(* Logix 5000 Rung export; software revision 16.03 *)

MODULES
   MCMR : vendor None type None code None
   Remote_ENBT : vendor None type None code None
END_MODULES

TYPE MCMRInitOutputData :   // Used to bring the Module into a known state after a restart operation.
STRUCT
   InitOutBlkIDLim : INT;   // Block Index Limit for ReadData size of the array
END_STRUCT
END_TYPE

TYPE MCMRCmdControl :   // Tags for command control
STRUCT
   CmdTrigger : BOOL;   // Command Trigger
   CmdControlData : INT[21];   // Command Control Data
   CmdControlResp : INT[5];   // Command Control Response
   CmdErrTrigger : BOOL;   // Command Error Trigger
   CmdErrData : INT[102];   // Command Error Data
END_STRUCT
END_TYPE

TYPE MCMRDATA :   // This object contains the Read & Write Data Arrays.
STRUCT
   ReadData : INT[600];   // Data read from module
   WriteData : INT[600];   // Data to write to module
END_STRUCT
END_TYPE

TYPE MCMRUTIL :   // This object stores all the variables required for data transfer operation between the module and the controller.
STRUCT
   LastRead : INT;   // Index of last read block
   LastWrite : INT;   // Index of last write block
   BlockIndex : INT;   // Computed block offset for data table
   ReadDataSize : DINT;   // Size of Read Data Array
   WriteDataSize : DINT;   // Size of Write Data Array
   RBTSremainder : INT;   // Computed remainder from Read Data Array size
   WBTSremainder : INT;   // Computed remainder from Write Data Array size
   MaxReadBlock : DINT;   // Maximum read block
   MaxWriteBlock : DINT;   // Maximum write block
   InitOutputData : MCMRInitOutputData;   // This is to initialize output data module reads data from PLC
END_STRUCT
END_TYPE

TYPE MCMRModuleDef :   // This object contains variables to be used with the module and status data related to the module.
STRUCT
   DATA : MCMRDATA;   // Read Data and Write Data
   STATUS : MCMRSTATUS;   // Status information in each read block
   CONTROL : MCMRCONTROL;   // Command Control Object
   UTIL : MCMRUTIL;   // Backplane Object
END_STRUCT
END_TYPE

TYPE MCMRSTATUS :   // This status data is returned on each read block and can be used to detect proper module operation.
STRUCT
   PassCnt : INT;   // Program cycle counter
   Product : INT[2];   // Product Name
   Rev : INT[2];   // Revision Level Number
   OP : INT[2];   // Operating Level Number
   Run : INT[2];   // Run Number
   Port1Stats : MCMRPortStats;   // Port error statistics for Port 1
   Port2Stats : MCMRPortStats;   // Port error statistics for Port 2
   Block : MCMRBlockStats;   // Block transfer statistics
   Port1CurrentErr : INT;   // Current error/index for Port 1
   Port1LastErr : INT;   // Last error/index for Port 1
   Port2CurrentErr : INT;   // Current error/index for Port 2
   Port2LastErr : INT;   // Last error/index for Port 2
   StatusMsgData : INT[46];   // Triggers status message data
   StatusTrigger : BOOL;   // Triggers Status reading.
END_STRUCT
END_TYPE

TYPE MCMRCONTROL :   // Tags used for special blocks
STRUCT
   ColdBoot : BOOL;   // Cold Boot
   WarmBoot : BOOL;   // Warm Boot
   CmdControlP1 : MCMRCmdControl;   // Command Control for Port 1
   CmdControlP2 : MCMRCmdControl;   // Command Control for Port 2
   EventTriggerP1 : BOOL;   // Triggers the Event Command.
   EventTriggerP2 : BOOL;   // Triggers the Event Command.
   EventCmdP1 : MCMREventCmd[100];   // Event Command for Port 1
   EventCmdP2 : MCMREventCmd[100];   // Event Command for Port 2
   EventCmdRespP1 : INT[5];   // Event Command Response for Port 1
   EventCmdRespP2 : INT[5];   // Event Command Response for Port 2
END_STRUCT
END_TYPE

TYPE MCMREventCmd :   // This object is used to contain the attributes to define a master command. An array of these objects is used for each port.
STRUCT
   Enable : INT;   // 0=Disable,1=Continuous,2=Event Command
   IntAddress : INT;   // Module's internal address associated with the command
   PollInt : INT;   // Minimum number of seconds between issuance of command (0-65535 Sec)
   Count : INT;   // Number of registers associated with the command
   Swap : INT;   // Swap code used with command
   Device : INT;   // Device index in Device Table to associate with the command
   Func : INT;   // Function code for the command
   DevAddress : INT;   // Address in device associated with the command
END_STRUCT
END_TYPE

TYPE MCMRPortStats :   // This object is used to store the port statistics
STRUCT
   PortTrigger : BOOL;   // Triggers port status reading
   CmdReq : INT;   // Total number of command list requests sent
   CmdResp : INT;   // Total number of command list responses received
   CmdErr : INT;   // Total number of command list errors
   Requests : INT;   // Total number of requests for port
   Responses : INT;   // Total number of responses for port
   ErrSent : INT;   // Total number of errors sent
   ErrRec : INT;   // Total number of errors received
   SlaveStats : SINT[250];   // Port Slave status values
END_STRUCT
END_TYPE

TYPE MCMRBlockStats :   // This object is used to store the block transfer statistics for the module.
STRUCT
   Read : INT;   // Total number of read block transfers
   Write : INT;   // Total number of write block transfers
   Parse : INT;   // Total number of blocks parsed
   Event : INT;   // Total number of event blocks received
   Cmd : INT;   // Total number of command blocks received
   Err : INT;   // Total number of block transfer errors
END_STRUCT
END_TYPE

ADD_ON_INSTRUCTION AOI56MCMR   (* revision 1.5, vendor ProSoft Technology Inc., ExecutePrescan *)
// Add-On - MVI56-MCMR & MVI56E-MCMR modules.
// Revision note:
// v1.5 - Initialize output data block now flexible to accommodate for flexible read and write data arrays.
VAR_IN_OUT
   Connection_Input : INT[42]; {required}   // Input parameters.
   Connection_Output : INT[42]; {required}   // Output parameters.
   MCMR : MCMRModuleDef; {required}
   CmdControlP1_MSG : MESSAGE; {required}
   CmdControlP2_MSG : MESSAGE; {required}
   CmdControlRespP1_MSG : MESSAGE; {required}
   CmdControlRespP2_MSG : MESSAGE; {required}
   CmdErrorP1_MSG : MESSAGE; {required}
   CmdErrorP2_MSG : MESSAGE; {required}
   EventCmdP1_MSG : MESSAGE; {required}
   EventCmdP2_MSG : MESSAGE; {required}
   EventCmdRespP1_MSG : MESSAGE; {required}
   EventCmdRespP2_MSG : MESSAGE; {required}
   SlaveStatusP1_MSG : MESSAGE; {required}
   SlaveStatusP2_MSG : MESSAGE; {required}
   ModuleStatus_MSG : MESSAGE; {required}
END_VAR
VAR
   MJFAULTS : DINT[12];
END_VAR

ROUTINE Logic   (* ladder *)
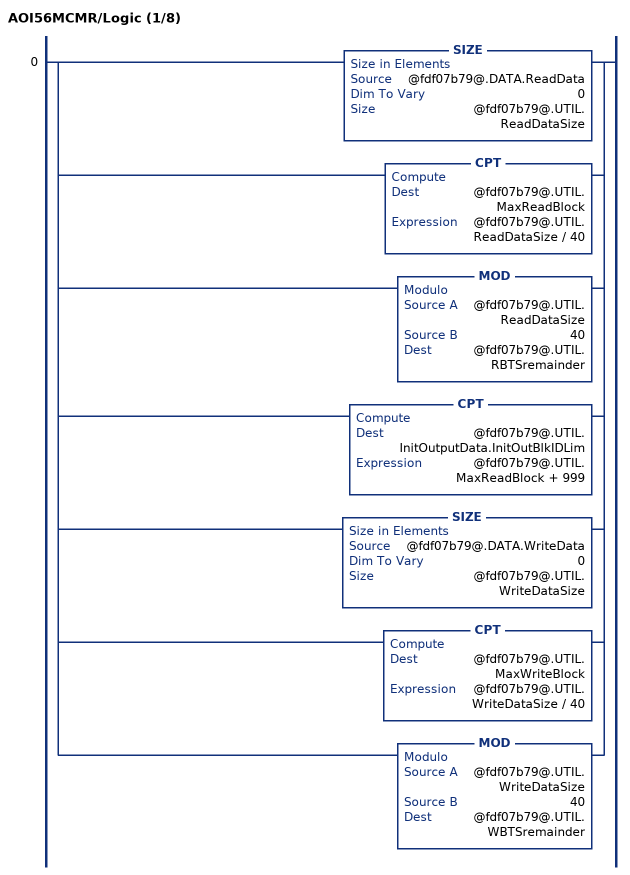
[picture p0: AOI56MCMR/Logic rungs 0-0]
   0: [SIZE(@fdf07b79@.DATA.ReadData,0,@fdf07b79@.UTIL.ReadDataSize) ,CPT(@fdf07b79@.UTIL.MaxReadBlock,@fdf07b79@.UTIL.ReadDataSize / 40) ,MOD(@fdf07b79@.UTIL.ReadDataSize,40,@fdf07b79@.UTIL.RBTSremainder) ,CPT(@fdf07b79@.UTIL.InitOutputData.InitOutBlkIDLim,@fdf07b79@.UTIL.MaxReadBlock + 999) ,SIZE(@fdf07b79@.DATA.WriteData,0,@fdf07b79@.UTIL.WriteDataSize) ,CPT(@fdf07b79@.UTIL.MaxWriteBlock,@fdf07b79@.UTIL.WriteDataSize / 40) ,MOD(@fdf07b79@.UTIL.WriteDataSize,40,@fdf07b79@.UTIL.WBTSremainder) ];
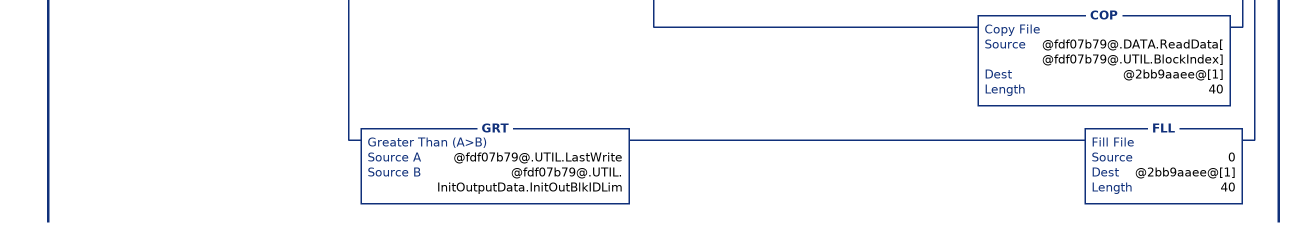
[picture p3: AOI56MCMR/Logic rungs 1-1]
   // This rung is used to check for a new read block from the MVI56-MBP module in slot 1.  If new data is available, the LastRead and word[0] will not be equal.  This will force the program to call the ReadData subroutine to process the new data received.  After the new data is placed in the Modbus Data Table, the program will send new data to the module using the WriteData subroutine.
   1: NEQ(@de25fda7@[41],@fdf07b79@.UTIL.LastRead)[MOV(@de25fda7@[41],@fdf07b79@.UTIL.LastRead) ,GEQ(@fdf07b79@.UTIL.LastRead,1) [LEQ(@fdf07b79@.UTIL.LastRead,@fdf07b79@.UTIL.MaxReadBlock) [CPT(@fdf07b79@.UTIL.BlockIndex,(@fdf07b79@.UTIL.LastRead - 1) * 40) ,COP(@de25fda7@[1],@fdf07b79@.DATA.ReadData[@fdf07b79@.UTIL.BlockIndex],40) ] ,CMP(@fdf07b79@.UTIL.LastRead - @fdf07b79@.UTIL.MaxReadBlock = 1) GRT(@fdf07b79@.UTIL.RBTSremainder,0) [CPT(@fdf07b79@.UTIL.BlockIndex,(@fdf07b79@.UTIL.LastRead - 1) * 40) ,COP(@de25fda7@[1],@fdf07b79@.DATA.ReadData[@fdf07b79@.UTIL.BlockIndex],@fdf07b79@.UTIL.RBTSremainder) ] ] ,MOV(@de25fda7@[0],@fdf07b79@.UTIL.LastWrite) ,XIC(@fdf07b79@.CONTROL.WarmBoot) [MOV(9998,@fdf07b79@.UTIL.LastWrite) ,MOV(9998,@2bb9aaee@[0]) ,OTU(@fdf07b79@.CONTROL.WarmBoot) ] ,XIC(@fdf07b79@.CONTROL.ColdBoot) [MOV(9999,@fdf07b79@.UTIL.LastWrite) ,MOV(9999,@2bb9aaee@[0]) ,OTU(@fdf07b79@.CONTROL.ColdBoot) ] ,[EQU(-1,@fdf07b79@.UTIL.LastWrite) ,EQU(0,@fdf07b79@.UTIL.LastWrite) ] MOV(@fdf07b79@.UTIL.LastWrite,@2bb9aaee@[0]) ,GEQ(@fdf07b79@.UTIL.LastWrite,1) [LEQ(@fdf07b79@.UTIL.LastWrite,@fdf07b79@.UTIL.MaxWriteBlock) [CPT(@fdf07b79@.UTIL.BlockIndex,(@fdf07b79@.UTIL.LastWrite - 1) * 40) ,COP(@fdf07b79@.DATA.WriteData[@fdf07b79@.UTIL.BlockIndex],@2bb9aaee@[1],40) ] ,CMP(@fdf07b79@.UTIL.LastWrite - @fdf07b79@.UTIL.MaxWriteBlock = 1) GRT(@fdf07b79@.UTIL.WBTSremainder,0) [CPT(@fdf07b79@.UTIL.BlockIndex,(@fdf07b79@.UTIL.LastWrite - 1) * 40) ,COP(@fdf07b79@.DATA.WriteData[@fdf07b79@.UTIL.BlockIndex],@2bb9aaee@[1],@fdf07b79@.UTIL.WBTSremainder) ] ,MOV(@fdf07b79@.UTIL.LastWrite,@2bb9aaee@[0]) ] ,LIM(1000,@fdf07b79@.UTIL.LastWrite,1124) [LEQ(@fdf07b79@.UTIL.LastWrite,@fdf07b79@.UTIL.InitOutputData.InitOutBlkIDLim) [CPT(@fdf07b79@.UTIL.BlockIndex,(@fdf07b79@.UTIL.LastWrite - 1000) * 40) ,COP(@fdf07b79@.DATA.ReadData[@fdf07b79@.UTIL.BlockIndex],@2bb9aaee@[1],40) ] ,GRT(@fdf07b79@.UTIL.LastWrite,@fdf07b79@.UTIL.InitOutputData.InitOutBlkIDLim) FLL(0,@2bb9aaee@[1],40) ] ];
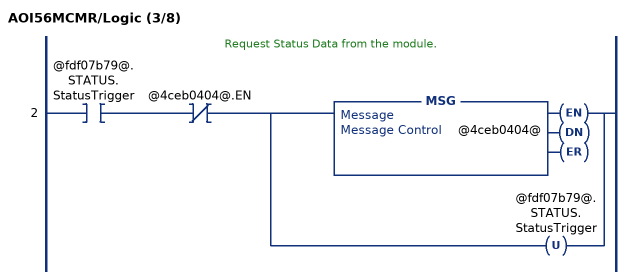
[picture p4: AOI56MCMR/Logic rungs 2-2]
   // Request Status Data from the module.
   2: XIC(@fdf07b79@.STATUS.StatusTrigger)XIO(@4ceb0404@.EN)[MSG(@4ceb0404@) ,OTU(@fdf07b79@.STATUS.StatusTrigger) ];
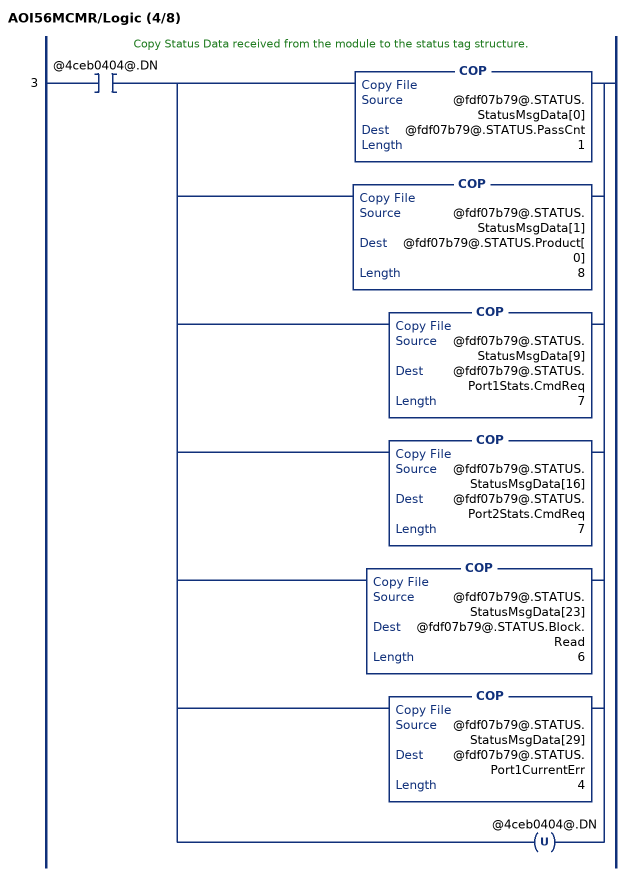
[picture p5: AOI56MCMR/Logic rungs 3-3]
   // Copy Status Data received from the module to the status tag structure.
   3: XIC(@4ceb0404@.DN)[COP(@fdf07b79@.STATUS.StatusMsgData[0],@fdf07b79@.STATUS.PassCnt,1) ,COP(@fdf07b79@.STATUS.StatusMsgData[1],@fdf07b79@.STATUS.Product[0],8) ,COP(@fdf07b79@.STATUS.StatusMsgData[9],@fdf07b79@.STATUS.Port1Stats.CmdReq,7) ,COP(@fdf07b79@.STATUS.StatusMsgData[16],@fdf07b79@.STATUS.Port2Stats.CmdReq,7) ,COP(@fdf07b79@.STATUS.StatusMsgData[23],@fdf07b79@.STATUS.Block.Read,6) ,COP(@fdf07b79@.STATUS.StatusMsgData[29],@fdf07b79@.STATUS.Port1CurrentErr,4) ,OTU(@4ceb0404@.DN) ];
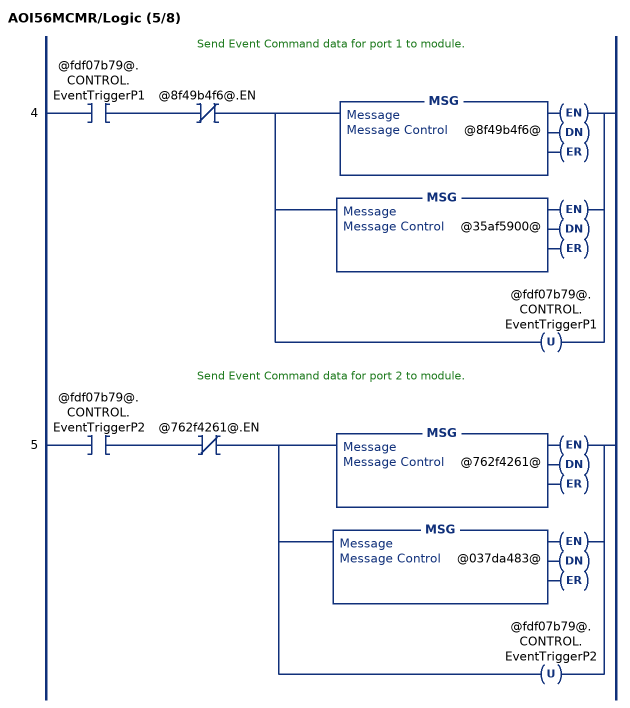
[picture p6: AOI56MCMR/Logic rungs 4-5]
   // Send Event Command data for port 1 to module.
   4: XIC(@fdf07b79@.CONTROL.EventTriggerP1)XIO(@8f49b4f6@.EN)[[MSG(@8f49b4f6@) ,MSG(@35af5900@) ] ,OTU(@fdf07b79@.CONTROL.EventTriggerP1) ];
   // Send Event Command data for port 2 to module.
   5: XIC(@fdf07b79@.CONTROL.EventTriggerP2)XIO(@762f4261@.EN)[[MSG(@762f4261@) ,MSG(@037da483@) ] ,OTU(@fdf07b79@.CONTROL.EventTriggerP2) ];
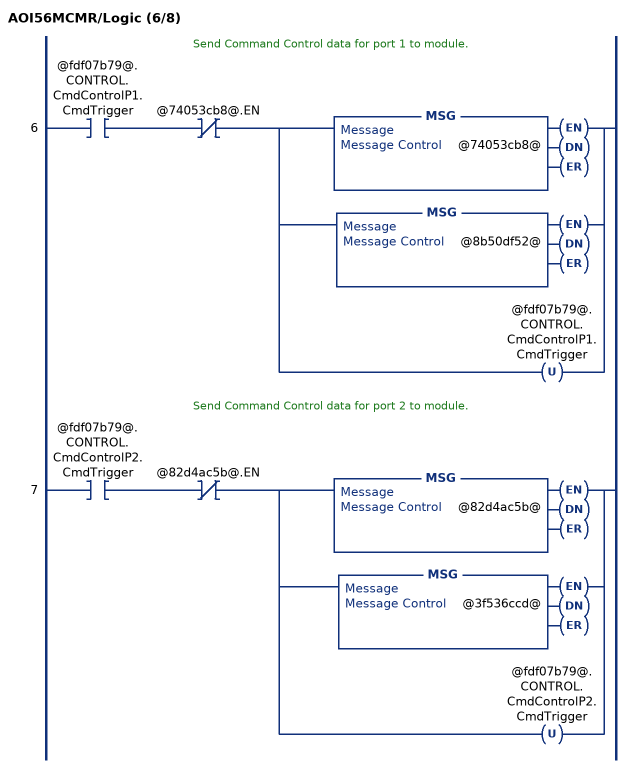
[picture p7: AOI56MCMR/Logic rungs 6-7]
   // Send Command Control data for port 1 to module.
   6: XIC(@fdf07b79@.CONTROL.CmdControlP1.CmdTrigger)XIO(@74053cb8@.EN)[[MSG(@74053cb8@) ,MSG(@8b50df52@) ] ,OTU(@fdf07b79@.CONTROL.CmdControlP1.CmdTrigger) ];
   // Send Command Control data for port 2 to module.
   7: XIC(@fdf07b79@.CONTROL.CmdControlP2.CmdTrigger)XIO(@82d4ac5b@.EN)[[MSG(@82d4ac5b@) ,MSG(@3f536ccd@) ] ,OTU(@fdf07b79@.CONTROL.CmdControlP2.CmdTrigger) ];
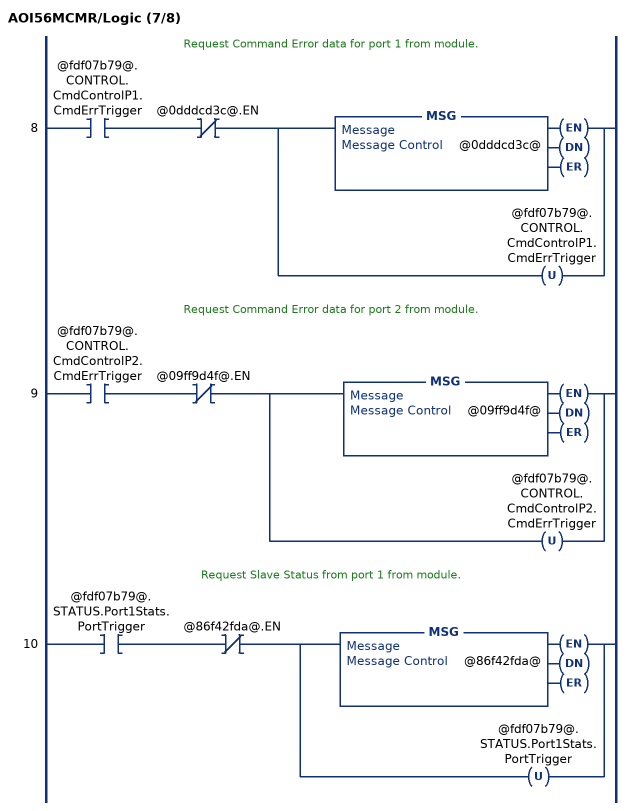
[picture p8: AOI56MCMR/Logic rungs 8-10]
   // Request Command Error data for port 1 from module.
   8: XIC(@fdf07b79@.CONTROL.CmdControlP1.CmdErrTrigger)XIO(@0dddcd3c@.EN)[MSG(@0dddcd3c@) ,OTU(@fdf07b79@.CONTROL.CmdControlP1.CmdErrTrigger) ];
   // Request Command Error data for port 2 from module.
   9: XIC(@fdf07b79@.CONTROL.CmdControlP2.CmdErrTrigger)XIO(@09ff9d4f@.EN)[MSG(@09ff9d4f@) ,OTU(@fdf07b79@.CONTROL.CmdControlP2.CmdErrTrigger) ];
   // Request Slave Status from port 1 from module.
   10: XIC(@fdf07b79@.STATUS.Port1Stats.PortTrigger)XIO(@86f42fda@.EN)[MSG(@86f42fda@) ,OTU(@fdf07b79@.STATUS.Port1Stats.PortTrigger) ];
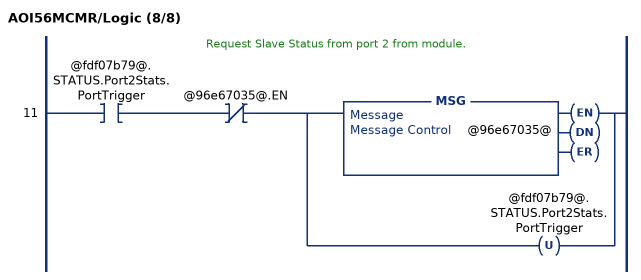
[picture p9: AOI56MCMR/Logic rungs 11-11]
   // Request Slave Status from port 2 from module.
   11: XIC(@fdf07b79@.STATUS.Port2Stats.PortTrigger)XIO(@96e67035@.EN)[MSG(@96e67035@) ,OTU(@fdf07b79@.STATUS.Port2Stats.PortTrigger) ];
END_ROUTINE

ROUTINE Prescan   (* ladder *)
// Startup
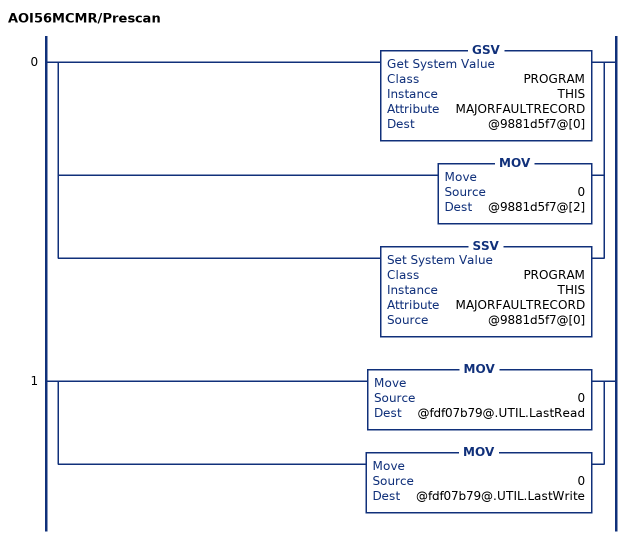
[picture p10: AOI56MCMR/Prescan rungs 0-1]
   0: [GSV(PROGRAM,THIS,MAJORFAULTRECORD,@9881d5f7@[0]) ,MOV(0,@9881d5f7@[2]) ,SSV(PROGRAM,THIS,MAJORFAULTRECORD,@9881d5f7@[0]) ];
   1: [MOV(0,@fdf07b79@.UTIL.LastRead) ,MOV(0,@fdf07b79@.UTIL.LastWrite) ];
END_ROUTINE
END_ADD_ON_INSTRUCTION

VAR_GLOBAL   (* controller tags *)
   CmdControlP2_MSG : MESSAGE;
        MessageParameters(MessageType := CIP Generic, RequestedLength := 42, ConnectedFlag := 2, ConnectionPath := MCMR, ServiceCode := 16#0010, ObjectType := 16#0004, TargetObject := 9912, AttributeNumber := 16#0003, LocalElement := MCMR.CONTROL.CmdControlP2.CmdControlData[0])
   CmdControlRespP1_MSG : MESSAGE;
        MessageParameters(MessageType := CIP Generic, ConnectedFlag := 2, ConnectionPath := MCMR, ServiceCode := 16#000e, ObjectType := 16#0004, TargetObject := 9902, AttributeNumber := 16#0003, DestinationTag := MCMR.CONTROL.CmdControlP1.CmdControlResp[0])
   EventCmdRespP1_MSG : MESSAGE;
        MessageParameters(MessageType := CIP Generic, ConnectedFlag := 2, ConnectionPath := MCMR, ServiceCode := 16#000e, ObjectType := 16#0004, TargetObject := 9901, AttributeNumber := 16#0003, DestinationTag := MCMR.CONTROL.EventCmdRespP1[0])
   CmdControlP1_MSG : MESSAGE;
        MessageParameters(MessageType := CIP Generic, RequestedLength := 42, ConnectedFlag := 2, ConnectionPath := MCMR, ServiceCode := 16#0010, ObjectType := 16#0004, TargetObject := 9902, AttributeNumber := 16#0003, LocalElement := MCMR.CONTROL.CmdControlP1.CmdControlData[0])
   Remote_ENBT:1:O : AB:1756_MODULE_INT_84Bytes:O:0;
   CmdErrorP1_MSG : MESSAGE;
        MessageParameters(MessageType := CIP Generic, ConnectedFlag := 2, ConnectionPath := MCMR, ServiceCode := 16#000e, ObjectType := 16#0004, TargetObject := 9950, AttributeNumber := 16#0003, DestinationTag := MCMR.CONTROL.CmdControlP1.CmdErrData[0])
   CmdErrorP2_MSG : MESSAGE;
        MessageParameters(MessageType := CIP Generic, ConnectedFlag := 2, ConnectionPath := MCMR, ServiceCode := 16#000e, ObjectType := 16#0004, TargetObject := 9951, AttributeNumber := 16#0003, DestinationTag := MCMR.CONTROL.CmdControlP2.CmdErrData[0])
   CmdControlRespP2_MSG : MESSAGE;
        MessageParameters(MessageType := CIP Generic, ConnectedFlag := 2, ConnectionPath := MCMR, ServiceCode := 16#000e, ObjectType := 16#0004, TargetObject := 9912, AttributeNumber := 16#0003, DestinationTag := MCMR.CONTROL.CmdControlP2.CmdControlResp[0])
   SlaveStatusP2_MSG : MESSAGE;
        MessageParameters(MessageType := CIP Generic, ConnectedFlag := 2, ConnectionPath := MCMR, ServiceCode := 16#000e, ObjectType := 16#0004, TargetObject := 9961, AttributeNumber := 16#0003, DestinationTag := MCMR.STATUS.Port2Stats.SlaveStats[0])
   AOI56MCMR : AOI56MCMR;
   Remote_ENBT:1:I : AB:1756_MODULE_INT_84Bytes:I:0;
   EventCmdRespP2_MSG : MESSAGE;
        MessageParameters(MessageType := CIP Generic, ConnectedFlag := 2, ConnectionPath := MCMR, ServiceCode := 16#000e, ObjectType := 16#0004, TargetObject := 9911, AttributeNumber := 16#0003, DestinationTag := MCMR.CONTROL.EventCmdRespP2[0])
   MCMR : MCMRModuleDef;
   ModuleStatus_MSG : MESSAGE;
        MessageParameters(MessageType := CIP Generic, ConnectedFlag := 2, ConnectionPath := MCMR, ServiceCode := 16#000e, ObjectType := 16#0004, TargetObject := 9250, AttributeNumber := 16#0003, DestinationTag := MCMR.STATUS.StatusMsgData[0])
   SlaveStatusP1_MSG : MESSAGE;
        MessageParameters(MessageType := CIP Generic, ConnectedFlag := 2, ConnectionPath := MCMR, ServiceCode := 16#000e, ObjectType := 16#0004, TargetObject := 9960, AttributeNumber := 16#0003, DestinationTag := MCMR.STATUS.Port1Stats.SlaveStats[0])
   EventCmdP2_MSG : MESSAGE;
        MessageParameters(MessageType := CIP Generic, RequestedLength := 20, ConnectedFlag := 2, ConnectionPath := MCMR, ServiceCode := 16#0010, ObjectType := 16#0004, TargetObject := 9911, AttributeNumber := 16#0003, LocalElement := MCMR.CONTROL.EventCmdP2[0])
   EventCmdP1_MSG : MESSAGE;
        MessageParameters(MessageType := CIP Generic, RequestedLength := 20, ConnectedFlag := 2, ConnectionPath := MCMR, ServiceCode := 16#0010, ObjectType := 16#0004, TargetObject := 9901, AttributeNumber := 16#0003, LocalElement := MCMR.CONTROL.EventCmdP1[0])
END_VAR

PROGRAM MainProgram

ROUTINE MainRoutine   (* ladder *)
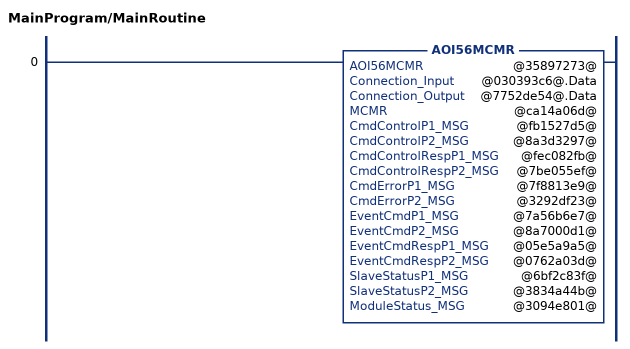
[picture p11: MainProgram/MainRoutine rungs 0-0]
   0: AOI56MCMR(@35897273@,@030393c6@.Data,@7752de54@.Data,@ca14a06d@,@fb1527d5@,@8a3d3297@,@fec082fb@,@7be055ef@,@7f8813e9@,@3292df23@,@7a56b6e7@,@8a7000d1@,@05e5a9a5@,@0762a03d@,@6bf2c83f@,@3834a44b@,@3094e801@);
END_ROUTINE
END_PROGRAM
